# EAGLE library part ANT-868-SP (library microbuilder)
SMT Antenna Antenna Factor 868MHz (1.10"x0.54") - Digikey: ANT-868-SP_-ND
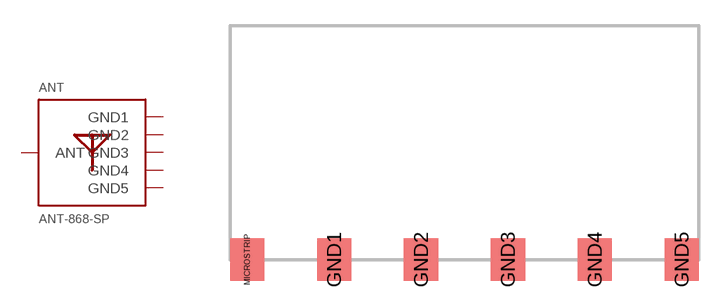
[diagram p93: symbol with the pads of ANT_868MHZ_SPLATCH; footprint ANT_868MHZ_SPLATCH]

Designator prefix ANT

## ANT-868-SP  [ANT_868MHZ_SPLATCH]
GND1  GND1  pwr
GND2  GND2  pwr
GND3  GND3  pwr
GND4  GND4  pwr
GND5  GND5  pwr
MICROSTRIP  ANT

## Footprint ANT_868MHZ_SPLATCH (pad centres in mm)
smd 2 x 2.5: GND1 -7.62,0; GND2 -2.54,0; GND3 2.54,0; GND4 7.62,0; GND5 12.7,0; MICROSTRIP -12.7,0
